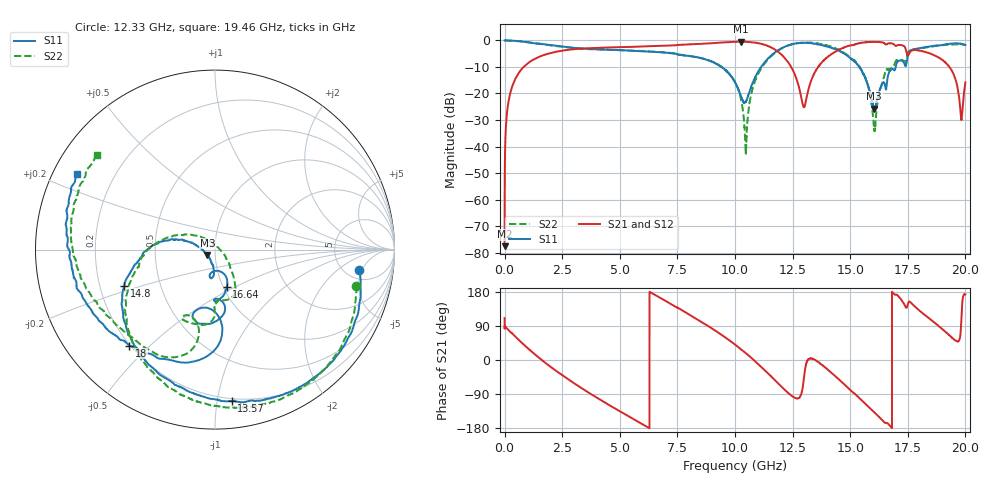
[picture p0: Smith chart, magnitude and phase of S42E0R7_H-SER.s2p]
!{S42E0R7}
!Johanson Technology Inc.
!www.johansontechnology.com
!Test Board Conditions:
!Substrate Type  RO4350B
!Substrate Thickness  50 mil
!Substrate Dk  3.66
!TL Type: GCPW
!TL Trace Width  60 mil
!TL Gap  10 mil
!Electrode orientation  Horizontal
!DUT TOPOLOGY	SERIES
!Mounting Pad LxW  14x55 mil
! Created Wed Nov 25 21:27:26 2020
# khz S ma R 50
! 2 Port Network Data from SP1.SP block
! freq  magS11  angS11  magS21  angS21  magS12  angS12  magS22  angS22
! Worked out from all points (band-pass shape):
!   20001 points, 300 kHz to 20 GHz, reference 50 ohm
!   highest |S21| = -0.47 dB at 10.26 GHz (marker M1); lowest = -77.6 dB at 300 kHz (marker M2)
!   |S21| within 3 dB of the highest: 2.821 GHz to 11.74 GHz (8.916 GHz wide, 122 % of centre); 14.52 GHz to 17.42 GHz (2.898 GHz wide, 18.2 % of centre)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
!   lowest |S11| = -25.7 dB at 16.04 GHz (marker M3), VSWR 1.11, Z = 45.9 - j2.8 ohm
!   |S11| at or under -10 dB: 9.409 GHz to 11.13 GHz (1.725 GHz wide, 16.8 % of centre); 11.13476 GHz to 11.13535 GHz (590 kHz wide, 0.0053 % of centre); 15.39 GHz to 16.98 GHz (1.581 GHz wide, 9.77 % of centre)
!   |S22| runs from -42.6 to 0.0 dB; largest |S21 - S12| = 0.02
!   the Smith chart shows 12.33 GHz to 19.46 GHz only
!   S11 on the Smith chart (normalised r, x): 12.33 GHz: 6.59, -4.41; 13.57 GHz: 0.18, -1.10; 14.8 GHz: 0.31, -0.17; 16.64 GHz: 1.04, -0.45; 18 GHz: 0.20, -0.43; 19.46 GHz: 0.07, +0.26
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300  0.9988 -0.2  0.0001323 110.6  0.0001929 62.1  1 -0.3
133300  0.9975 -8.1  0.05528 81.5  0.05555 81.4  0.9983 -8.1
510300  0.9773 -31.1  0.2056 59.2  0.2064 59.3  0.978 -30.9
1622300  0.8556 -90.2  0.5166 -0.4  0.5172 -0.5  0.8517 -90.9
3334300  0.7067 -165.5  0.7009 -74.0  0.7006 -74.0  0.7039 -162.4
6667300  0.6021 82.6  0.79 166.9  0.7881 166.8  0.6078 72.3
1.00003e7  0.1624 -36.9  0.9422 40.8  0.9428 40.9  0.1641 -49.4
1.02593e7  0.08942 -24.1  0.9475 28.6  0.9458 28.6  0.07777 -66.8
1.04763e7  0.07127 27.5  0.9414 17.8  0.9424 17.8  0.008482 175.6
1.10093e7  0.2599 57.2  0.8882 -10.7  0.8863 -10.5  0.2349 74.9
1.23313e7  0.8111 -8.1  0.3744 -88.3  0.3791 -87.7  0.8113 -14.6
1.29773e7  0.9044 -47.1  0.05553 -54.8  0.05611 -55.4  0.91 -54.3
1.33343e7  0.8852 -69.5  0.1881 3.8  0.1887 3.3  0.9007 -74.6
1.35683e7  0.8492 -83.7  0.2982 -3.5  0.2971 -3.9  0.8803 -87.4
1.48003e7  0.5433 -158.2  0.7589 -67.4  0.7569 -67.6  0.5652 -151.7
1.60443e7  0.05199 -144.1  0.9392 -138.0  0.9392 -137.9  0.02046 59.5
1.66413e7  0.2168 -72.6  0.8732 -167.9  0.8662 -168.2  0.2803 -84.4
1.66673e7  0.2357 -75.6  0.8834 -169.7  0.8724 -170.1  0.2819 -85.9
1.80013e7  0.7165 -131.8  0.6428 130.6  0.6499 131.7  0.6962 -146.2
1.94623e7  0.8797 151.0  0.2438 56.9  0.2471 56.2  0.8436 141.2
1.98093e7  0.8609 129.2  0.03555 86.8  0.03575 87.0  0.8455 115.0
2e7  0.823 114.7  0.1617 173.2  0.1635 173.9  0.8075 98.3
